(* Logix 5000 AddOnInstructionDefinition export CM1T_WriteRegister; software revision 20.00 *)

TYPE CM1T_DriveStatus :
STRUCT
   StatusValue : SINT;   // Indicates status and error type
   StatusValue1 : SINT;   // Additional status values
   In_Position : BOOL;   // Drive is in position and ready to move
   Moving : BOOL;   // Drive is currently moving
   Disabled : BOOL;   // Drive is disabled
   Error : BOOL;   // Drive is in an error state
   MoveComplete : BOOL;   // Move Complete
   NewStartRequired : BOOL;   // New setpoint required
   HomeAchieved : BOOL;   // Home achieved
END_STRUCT
END_TYPE

TYPE CM1T_Controlword :
STRUCT
   Start : BOOL;   // Start a motion or set a new setpoint
   Halt : BOOL;   // Halt the current motion
   Relative_Move : BOOL;   // Execute the position profile as a relative move
   Speed_Control : BOOL;   // Execute the profile as speed control only
   Disable : BOOL;   // Disable the drive (zero torque)
   Reset_Error : BOOL;   // Reset any existing errors with rising edge
   Set_to_Zero : BOOL;   // Set the current position to 0
   Home : BOOL;   // Execute a home search
END_STRUCT
END_TYPE

TYPE CM1T_Axis :
STRUCT
   Input : SINT[36];   // Data coming from the CM1-T
   Output : SINT[28];   // Data going to the CM1-T
   us50Counter : DINT;   // Controller 50us counter
   ModeOfOperation : SINT;   // Type of motion control mode
   ModeOfOperationDisplay : SINT;   // Indicates the active control mode
   Controlword : CM1T_Controlword;   // Controls the drive operation
   DriveStatus : CM1T_DriveStatus;   // Shows status of the drive
   PositionTarget : DINT;   // Final target position for position move
   SpeedTarget : DINT;   // Maximum speed for target move
   TorqueTarget : INT;   // Max torque allowed in 0.1% of peak. Typically 1100
   AccelerationTarget : INT;   // Acceleration for profile move
   DecelerationTarget : INT;   // Deceleration for profile move
   PositionActual : DINT;   // Actual position of the drive
   TargetActual : DINT;   // 1ms position target
   PositionError : DINT;   // Error between the current drive position and the instantaneous target position
   SpeedActual : DINT;   // Actual speed of the drive
   CurrentActual : INT;   // 0.1% of rated current
   OverloadActual : INT;   // 0.1% of overload torque
   DCVoltage : INT;   // DC voltage bus. 0.1V unit
   AnalogIN : INT;   // Value of 10bit analog input
   DigitalIN : SINT;   // Read the digital inputs
   DigitalOUT : SINT;   // Set the digital outputs
   Temperature : SINT;   // Temperature of the drive
   ErrorCode : SINT;   // Indicates error in Ethernet/IP module
   ReadAddress1 : INT;   // Read Address 1
   ReadValue1 : DINT;   // Value read from register
   ReadValueAddress1 : INT;   // Responding register address
   WriteValue1 : DINT;   // Value to write
   WriteAddress1 : INT;   // Write Address 1
END_STRUCT
END_TYPE

ADD_ON_INSTRUCTION CM1T_WriteRegister   (* revision 1.0 *)
// WriteRegister
VAR_IN_OUT
   CM1T_Axis : CM1T_Axis; {required}
END_VAR
VAR_INPUT
   Address : INT; {required}
   Value : DINT; {access Read Only, required}
END_VAR
VAR_OUTPUT
   Done : BOOL; {access Read Only, visible}
END_VAR
VAR
   usCount : DINT; {access None}
END_VAR

ROUTINE Logic   (* ladder *)
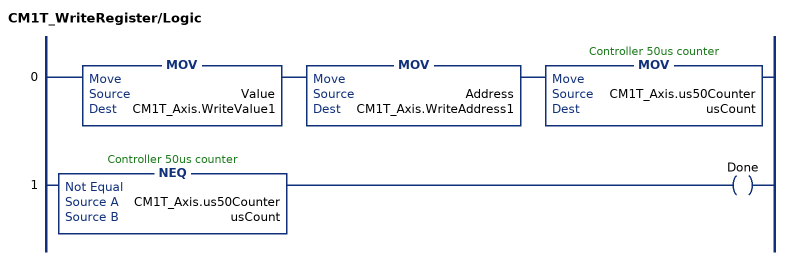
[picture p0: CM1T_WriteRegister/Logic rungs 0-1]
   0: MOV(Value,CM1T_Axis.WriteValue1)MOV(Address,CM1T_Axis.WriteAddress1)MOV(CM1T_Axis.us50Counter,usCount);
   1: NEQ(CM1T_Axis.us50Counter,usCount)OTE(Done);
END_ROUTINE
END_ADD_ON_INSTRUCTION
